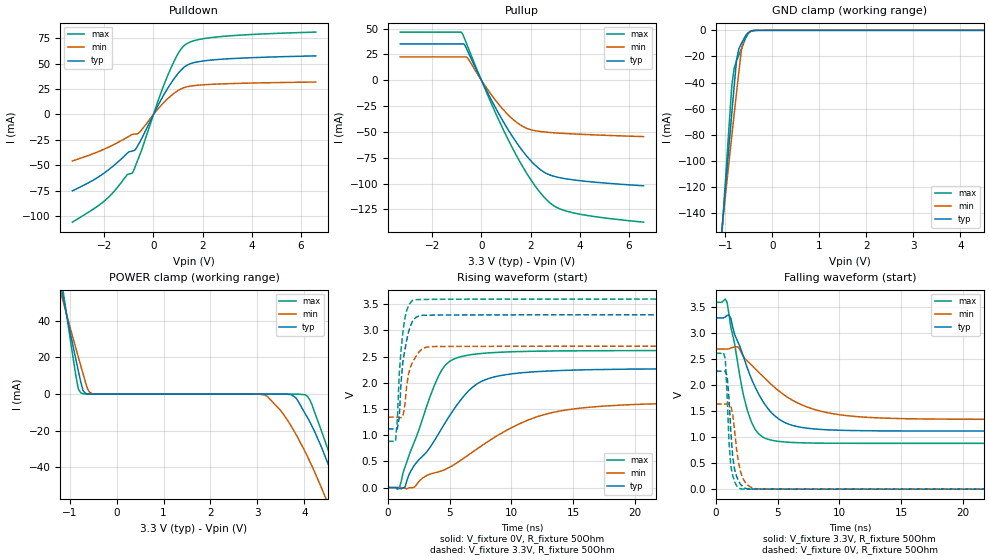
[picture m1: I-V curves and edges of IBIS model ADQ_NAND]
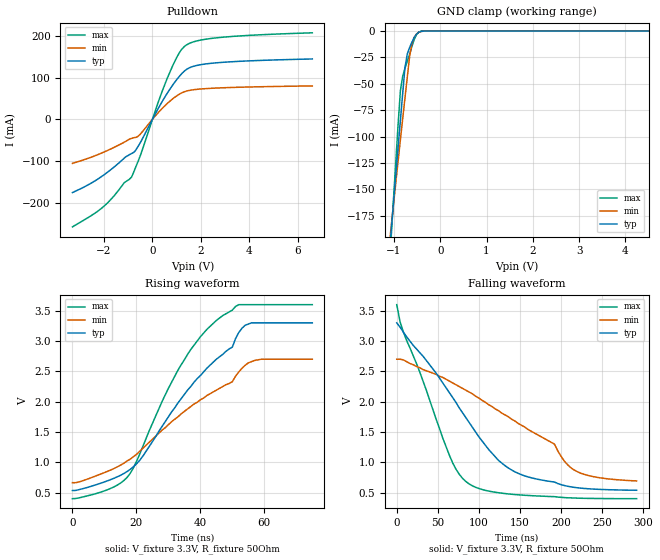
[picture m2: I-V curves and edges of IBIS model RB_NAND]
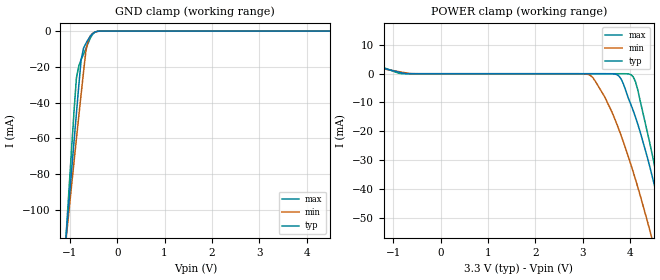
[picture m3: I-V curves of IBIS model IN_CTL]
| This IBIS file was created by s2ibis3 version 1.1
| North Carolina State University, ERL, 2006
[IBIS ver] 3.2
[File name] s34ml04g1_b_i_33_r3.ibs
[File Rev] 3.0
|   Rev1.0 Initial release (X16 ONFI F41 98462AB 41088)
|   Rev2.0 Regenerate RB model using 50Ohm R_fixture
|   & updated based on measurements
|   Rev3.0 Update 0A for 0V
[Date] 7/23/2014
[Source] Spansion IBIS team
|   Email: dl.ibisteam@spansion.com
[Notes]  Generated IBIS models from SPICE simulations.
|   VIO=3.3V, Temperature Range: Industrial (-40oC to +85oC).
[Disclaimer] THE MODEL LIBRARIES ARE PROVIDED AS IS.
[Copyright] (C) COPYRIGHT 2014
| SPANSION LLC
| ALL RIGHTS RESERVED.
|   Component S34ML04G1 X16 ONFI F41 in VBM063 package
[Component]   S34ML04G1
[Manufacturer]   Spansion
[Package]
| variable   typ   min   max
R_pkg   138.79mOhm   97.44mOhm   163.44mOhm
L_pkg   4.10nH   2.14nH   4.94nH
C_pkg   1.35pF   0.84pF   1.88pF
[Pin]   signal_name   model_name   R_pin   L_pin   C_pin
A1   R   NC
A2   R   NC
A9   R   NC
A10   R   NC
B1   R   NC
B9   R   NC
B10   R   NC
C3   WP#   IN_CTL   124.39m   4.65n   1.67p
C4   ALE   IN_CTL   97.44m   4.82n   1.88p
C5   VSS   GND
C6   CE#   IN_CTL   132.71m   4.06n   1.15p
C7   WE#   IN_CTL   147.28m   4.01n   1.31p
C8   RB#   RB_NAND   100.48m   2.14n   0.84p
D3   VDD   POWER
D4   RE#   IN_CTL   131.29m   4.44n   1.39p
D5   CLE   IN_CTL   135.91m   3.97n   1.34p
D6   R   NC
D7   R   NC
D8   R   NC
E3   R   NC
E4   R   NC
E5   R   NC
E6   R   NC
E7   R   NC
E8   R   NC
F3   R   NC
F4   R   NC
F5   R   NC
F6   R   NC
F7   VSS   GND
F8   R   NC
G3   R   NC
G4   VDD   POWER
G5   R   NC
G6   I/O13   ADQ_NAND   150.77m   4.57n   1.39p
G7   I/O15   ADQ_NAND   137.95m   3.52n   1.24p
G8   R   NC
H3   I/O8   ADQ_NAND   155.16m   4.94n   1.38p
H4   I/O0   ADQ_NAND   156.23m   4.28n   1.47p
H5   I/O10   ADQ_NAND   130.14m   3.86n   1.23p
H6   I/O12   ADQ_NAND   153.29m   4.44n   1.38p
H7   I/O14   ADQ_NAND   143.13m   3.57n   1.29p
H8   VDD   POWER
J3   I/O9   ADQ_NAND   143.73m   4.63n   1.83p
J4   I/O1   ADQ_NAND   132.18m   4.08n   1.16p
J5   I/O11   ADQ_NAND   123.32m   2.98n   1.14p
J6   VDD   POWER
J7   I/O5   ADQ_NAND   149.2m   3.93n   1.38p
J8   I/O7   ADQ_NAND   149.33m   4.06n   1.34p
K3   VSS   GND
K4   I/O2   ADQ_NAND   140.46m   4.3n   1.2p
K5   I/O3   ADQ_NAND   131.54m   3.7n   1.17p
K6   I/O4   ADQ_NAND   162.82m   4.85n   1.44p
K7   I/O6   ADQ_NAND   163.44m   4.41n   1.53p
K8   VSS   GND
L1   R   NC
L2   R   NC
L9   R   NC
L10   R   NC
M1   R   NC
M2   R   NC
M9   R   NC
M10   R   NC
| Models and submodels in the file (3): ADQ_NAND (I/O), RB_NAND (Open_drain), IN_CTL (Input)
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|   MODEL : ADQ_NAND
[Model]   ADQ_NAND
Model_type   I/O
Polarity   Non-Inverting
Enable   Active-High
Vinl   =  0.66V
Vinh   =  2.64V
Vmeas   =  1.65V
| variable   typ   min   max
C_comp   3.72pF   3.35pF   4.46pF
[Pullup Reference]   3.3V   2.7V   3.6V
[Pulldown Reference]   0V   0V   0V
[POWER Clamp Reference]  3.3V   2.7V   3.6V
[GND Clamp Reference]   0V   0V   0V
[Temperature Range]   25   85   -40
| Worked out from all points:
|   slope of the pulldown table from 0 to 0.495 V, typ, clamps not added: 22.1 ohm
|   slope of the pullup table from 0 to 0.495 V, typ, clamps not added: 21.4 ohm
|   GND clamp passes 1 mA (typ) near -0.48 V on its own axis
|   POWER clamp passes 1 mA (typ) near -0.68 V on its own axis
|   rising waveform, V_fixture 0V, R_fixture 50Ohm: 20-80 % time 4.19ns typ, 7.08ns min, 2.46ns max; typ from 0 V to 2.27 V
|   rising waveform, V_fixture 3.3V, R_fixture 50Ohm: 20-80 % time 603ps typ, 695ps min, 475ps max; typ from 1.12 V to 3.3 V
|   falling waveform, V_fixture 3.3V, R_fixture 50Ohm: 20-80 % time 2.48ns typ, 4.32ns min, 1.41ns max; typ from 3.3 V to 1.12 V
|   falling waveform, V_fixture 0V, R_fixture 50Ohm: 20-80 % time 430ps typ, 585ps min, 338ps max; typ from 2.27 V to 0 V
[GND Clamp]
| Voltage   I(typ)   I(min)   I(max)
-3.3V     -1.197A    -993.5mA   -1.473A
-1.111V   -168.7mA   -165.1mA   -177mA
-1.061V   -147.3mA   -148mA     -149.5mA
-862.3mV  -63mA      -80.53mA   -42.06mA
-812.6mV  -42.45mA   -64.03mA   -28.91mA
-762.8mV  -22.94mA   -47.74mA   -23.25mA
-713.1mV  -14.14mA   -31.74mA   -18.95mA
-663.3mV  -10.25mA   -16.14mA   -14.74mA
-613.6mV  -6.949mA   -7.536mA   -10.01mA
-563.8mV  -4.042mA   -3.753mA   -5.672mA
-464.3mV  -720.5uA   -733.4uA   -815.2uA
6.6V      1.359nA    6.676nA    724.9pA
[POWER Clamp]
| Voltage   I(typ)   I(min)   I(max)
-3.3V     375.4mA    292.7mA    492.2mA
-1.161V   55.92mA    52.85mA    60.54mA
-1.111V   49.46mA    48.02mA    51.76mA
-812.6mV  12.65mA    20.18mA    2.785mA
-713.1mV  1.991mA    11.14mA    210.2uA
-514.1mV  3.635uA    206.1uA    175.7nA
3.167V    -346.7pA   -651.9uA   -347pA
3.715V    -264.2uA   -17.29mA   -3.748nA
4.013V    -10.55mA   -31.37mA   -349.7uA
4.361V    -28.86mA   -51.02mA   -19.97mA
4.759V    -56.42mA   -77.19mA   -52.14mA
6.6V      -230mA     -237.7mA   -254.4mA
[Pulldown]
| Voltage   I(typ)   I(min)   I(max)
-3.3V     -74.86mA   -45.6mA    -105.6mA
-2.056V   -58.33mA   -34.54mA   -86.04mA
-1.609V   -49.97mA   -29.43mA   -75.64mA
-1.061V   -37.9mA    -22.31mA   -58.8mA
-862.3mV  -35.82mA   -19.52mA   -57.47mA
-613.6mV  -29.56mA   -18.54mA   -43.2mA
530.7mV   23.79mA    14.41mA    35.41mA
978.4mV   39.6mA     23.2mA     58.73mA
1.277V    47.02mA    26.66mA    68.18mA
1.725V    51.29mA    28.51mA    72.88mA
2.62V     53.95mA    29.87mA    76.16mA
6.6V      57.49mA    31.83mA    80.84mA
[Pullup]
| Voltage   I(typ)   I(min)   I(max)
-3.3V     35.11mA    22.59mA    46.56mA
-812.6mV  35.11mA    22.59mA    46.56mA
-713.1mV  35.11mA    22.59mA    41.95mA
-563.8mV  28.48mA    21.71mA    32.95mA
431.2mV   -20.24mA   -14.89mA   -23.98mA
1.277V    -54.95mA   -37.75mA   -66.24mA
1.675V    -68.41mA   -44.63mA   -83.44mA
2.123V    -80.74mA   -48.58mA   -100.2mA
2.521V    -88.55mA   -49.96mA   -112.4mA
2.869V    -92.39mA   -50.72mA   -120.2mA
3.864V    -96.8mA    -52.14mA   -129mA
6.6V      -102.2mA   -54.58mA   -137.4mA
[Ramp]
R_load   =  50Ohm
| variable   typ   min   max
dV/dt_r   1.3626/4.1889n   0.9774/7.0763n   1.5702/2.4557n
dV/dt_f   1.3080/2.4770n   0.8130/4.3173n   1.6304/1.4077n
|Slew_r   0.3253V/ns   0.1381V/ns   0.6394V/ns
|Slew_f   0.5281V/ns   0.1883V/ns   1.1582V/ns
[Rising Waveform]
V_fixture   =  0V
V_fixture_min   =  0V
V_fixture_max   =  0V
R_fixture   =  50Ohm
L_fixture   =  0H
C_fixture   =  0F
| Time   V(typ)   V(min)   V(max)
0s        0V         0V         0V
904.5ps   -17.81mV   243.6uV    -11.48mV
1.357ns   -1.281mV   -12.59mV   378.6mV
2.111ns   417.9mV    4.357mV    859.7mV
3.92ns    959.4mV    288.8mV    2.04V
4.673ns   1.254V     349.7mV    2.346V
5.578ns   1.575V     471mV      2.477V
7.99ns    2.069V     861.5mV    2.569V
13.57ns   2.231V     1.445V     2.609V
30ns      2.271V     1.629V     2.617V
[Rising Waveform]
V_fixture   =  3.3V
V_fixture_min   =  2.7V
V_fixture_max   =  3.6V
R_fixture   =  50Ohm
L_fixture   =  0H
C_fixture   =  0F
| Time   V(typ)   V(min)   V(max)
0s        1.12V      1.345V     882.6mV
603ps     1.119V     1.345V     881.7mV
753.8ps   1.12V      1.344V     1.297V
904.5ps   1.335V     1.341V     2.16V
1.055ns   2.019V     1.332V     2.626V
1.206ns   2.411V     1.367V     2.984V
1.658ns   2.973V     2.17V      3.474V
1.96ns    3.167V     2.381V     3.571V
3.618ns   3.293V     2.693V     3.595V
30ns      3.3V       2.699V     3.6V
[Falling Waveform]
V_fixture   =  3.3V
V_fixture_min   =  2.7V
V_fixture_max   =  3.6V
R_fixture   =  50Ohm
L_fixture   =  0H
C_fixture   =  0F
| Time   V(typ)   V(min)   V(max)
0s        3.3V       2.7V       3.6V
904.5ps   3.347V     2.699V     3.593V
1.206ns   3.288V     2.718V     3.118V
1.809ns   2.821V     2.736V     2.36V
2.563ns   2.319V     2.463V     1.504V
3.166ns   1.972V     2.323V     1.156V
4.07ns    1.597V     2.111V     972.8mV
6.181ns   1.23V      1.716V     899.8mV
10.1ns    1.134V     1.431V     884mV
30ns      1.12V      1.345V     882.6mV
[Falling Waveform]
V_fixture   =  0V
V_fixture_min   =  0V
V_fixture_max   =  0V
R_fixture   =  50Ohm
L_fixture   =  0H
C_fixture   =  0F
| Time   V(typ)   V(min)   V(max)
0s        2.273V     1.64V      2.617V
753.8ps   2.274V     1.64V      2.515V
904.5ps   2.182V     1.642V     1.795V
1.055ns   1.747V     1.641V     905.3mV
1.206ns   1.096V     1.595V     445.1mV
1.357ns   612.3mV    1.449V     264.2mV
1.508ns   383.6mV    1.133V     144.9mV
1.96ns    100.1mV    363.8mV    9.448mV
3.317ns   1.732mV    4.78mV     810.8uV
30ns      0V         -660.4nV   0V
|   MODEL : RB_NAND
[Model]   RB_NAND
Model_type   Open_drain
Polarity   Inverting
Enable   Active-High
Vref   = 3.300V
Vmeas   = 1.990V
Rref   = 50Ohm
| variable   typ   min   max
C_comp   3.28pF   3.22pF   3.30pF
[Pullup Reference]   3.3V   2.7V   3.6V
[Pulldown Reference]   0V   0V   0V
[POWER Clamp Reference]  3.3V   2.7V   3.6V
[GND Clamp Reference]   0V   0V   0V
[Temperature Range]   25   85   -40
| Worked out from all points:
|   slope of the pulldown table from 0 to 0.495 V, typ, clamps not added: 9.6 ohm
|   GND clamp passes 1 mA (typ) near -0.46 V on its own axis
|   rising waveform, V_fixture 3.3V, R_fixture 50Ohm: 20-80 % time 24.4ns typ, 30.1ns min, 18.2ns max; typ from 0.534 V to 3.3 V
|   falling waveform, V_fixture 3.3V, R_fixture 50Ohm: 20-80 % time 87.8ns typ, 131ns min, 52.9ns max; typ from 3.3 V to 0.539 V
[GND Clamp]
| Voltage   I(typ)   I(min)   I(max)
-3.3V     -1.508A    -1.227A    -1.955A
-1.061V   -189.3mA   -185.6mA   -195.8mA
-1.012V   -162.9mA   -164.8mA   -159.9mA
-862.3mV  -84.81mA   -103.2mA   -56.72mA
-812.6mV  -59.25mA   -83.1mA    -42.96mA
-762.8mV  -34.52mA   -63.26mA   -35.19mA
-713.1mV  -21.72mA   -43.7mA    -28.66mA
-663.3mV  -15.69mA   -24.3mA    -22.05mA
-613.6mV  -10.63mA   -11.92mA   -14.69mA
-563.8mV  -6.221mA   -5.981mA   -8.083mA
-464.3mV  -1.13mA    -1.178mA   -1.014mA
6.6V      1.358nA    7.86nA     604.8pA
[Pulldown]
| Voltage   I(typ)   I(min)   I(max)
-3.3V     -175.2mA   -105.3mA   -257.3mA
-2.056V   -135.2mA   -79.69mA   -210.9mA
-1.161V   -92.77mA   -54.55mA   -151.6mA
-862.3mV  -81.85mA   -45.48mA   -138.1mA
-514.1mV  -57.27mA   -36.28mA   -89.12mA
182.4mV   20.02mA    12.39mA    31.56mA
580.4mV   59.68mA    36.29mA    93.65mA
1.028V    97.03mA    57.28mA    151mA
1.327V    116mA      66.35mA    174.9mA
1.774V    128.4mA    71.55mA    187mA
2.57V     135.1mA    74.87mA    194.8mA
6.6V      144.7mA    80.15mA    207.3mA
[Ramp]
R_load   =  50Ohm
| variable   typ   min   max
dV/dt_r   1.6598/36.4373n   1.2358/41.5692n   1.9134/29.2836n
dV/dt_f   1.6550/32.9006n   1.2167/53.6425n   1.9127/21.1966n
|Slew_r   0.0456V/ns   0.0297V/ns   0.0653V/ns
|Slew_f   0.0503V/ns   0.0227V/ns   0.0902V/ns
[Rising Waveform]
V_fixture   =  3.3V
V_fixture_min   =  2.7V
V_fixture_max   =  3.6V
R_fixture   =  50Ohm
L_fixture   =  0H
C_fixture   =  0F
| Time   V(typ)   V(min)   V(max)
0s        534mV      664mV      400mV
11ns      696mV      852mV      549mV
17ns      845mV      1.02V      746mV
22ns      1.1V       1.23V      1.26V
33ns      1.98V      1.75V      2.52V
45ns      2.7V       2.19V      3.34V
50ns      2.9V       2.33V      3.51V
54ns      3.26V      2.6V       3.6V
59ns      3.3V       2.7V       3.6V
75ns      3.3V       2.7V       3.6V
[Falling Waveform]
V_fixture   =  3.3V
V_fixture_min   =  2.7V
V_fixture_max   =  3.6V
R_fixture   =  50Ohm
L_fixture   =  0H
C_fixture   =  0F
| Time   V(typ)   V(min)   V(max)
0s        3.3V       2.7V       3.6V
8ns       3.15V      2.69V      3.15V
64ns      2.15V      2.34V      1.12V
84ns      1.74V      2.19V      685mV
124ns     1.03V      1.85V      498mV
148ns     817mV      1.64V      464mV
192ns     675mV      1.3V       434mV
204ns     617mV      1.02V      418mV
220ns     580mV      844mV      409mV
292ns     539mV      693mV      400mV
|   MODEL : IN_CTL
[Model]   IN_CTL
Model_type   Input
Vinl   =  0.66V
Vinh   =  2.64V
| variable   typ   min   max
C_comp   2.20pF   1.98pF   2.64pF
[Pullup Reference]   3.3V   2.7V   3.6V
[Pulldown Reference]   0V   0V   0V
[POWER Clamp Reference]  3.3V   2.7V   3.6V
[GND Clamp Reference]   0V   0V   0V
[Temperature Range]   25   85   -40
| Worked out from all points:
|   GND clamp passes 1 mA (typ) near -0.50 V on its own axis
|   POWER clamp passes 1 mA (typ) near -1.00 V on its own axis
[GND Clamp]
| Voltage   I(typ)   I(min)   I(max)
-3.3V     -892.7mA   -757mA     -1.103A
-1.111V   -124.9mA   -124.4mA   -127.1mA
-1.061V   -108.9mA   -111.3mA   -106.1mA
-912.1mV  -61.44mA   -72.77mA   -44.48mA
-862.3mV  -45.92mA   -60.11mA   -26.21mA
-812.6mV  -30.62mA   -47.58mA   -19.53mA
-762.8mV  -16mA      -35.22mA   -15.96mA
-713.1mV  -9.615mA   -23.12mA   -12.96mA
-663.3mV  -6.937mA   -11.32mA   -9.972mA
-613.6mV  -4.694mA   -5.064mA   -6.639mA
-464.3mV  -475.4uA   -474.6uA   -451.8uA
6.6V      1.026nA    5.204nA    409.6pA
[POWER Clamp]
| Voltage   I(typ)   I(min)   I(max)
-3.3V     10.82mA    8.192mA    15.39mA
-862.3mV  458.5uA    653.2uA    96.2uA
3.118V    -137.7pA   -248.2uA   -142pA
3.466V    -116.3nA   -8.13mA    -146.7pA
3.764V    -796.7uA   -19.44mA   -14.44nA
4.013V    -10.55mA   -31.37mA   -275uA
4.113V    -15mA      -36.65mA   -2.721mA
4.162V    -17.51mA   -39.4mA    -5.6mA
4.411V    -31.97mA   -54.09mA   -23.68mA
4.759V    -56.42mA   -77.19mA   -53.17mA
4.809V    -60.24mA   -80.71mA   -57.87mA
6.6V      -230mA     -237.7mA   -258.8mA
